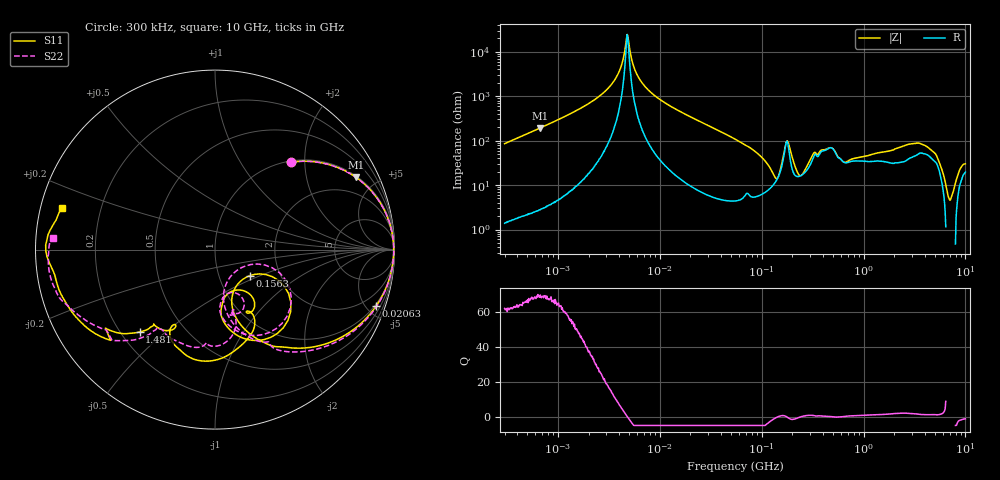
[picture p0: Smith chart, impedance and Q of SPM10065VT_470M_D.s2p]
! S-Parameter Data Generated by TDK Corporation
! Copyright(C) 2020 TDK Corporation.
! All Rights Reserved.
! TDK P/N: SPM10065VT-470M-D (Inductor)
! Property: L=47uH at 100kHz
! Size(LxWxT): 10.5x10x6.5mm
! Model Type: s2p (Touchstone File Format Version 1.0)
! Frequency: DC=Yes Start=0.3MHz Stop=10000MHz 802points Log-sweep
! Model Generated on Apr. 23, 2020
! Port Assignments:
!  1 ---@@@--- 2
! Applicable Conditions:
!  Temperature = 25 degC
!  DC Bias Current = 0 A
!  Small Signal Operation
! Terms and conditions regarding TDK Simulation Models
! (1)This simulation model is being provided solely for informational purposes. Please refer to the specifications of the products in terms of detailed characteristics of such products.
! (2)In no event shall TDK Corporation of any of its subsidiaries be liable for any loss or damage arising, directly or indirectly,
!  From any information contained in this simulation model, including, but not limited to loss or damages arising from any inaccuracies, omissions or errors in connection with such information.
! (3)Any and all copyrights on this simulation model are owned by TDK Corporation.
!  Duplication or redistribution of this simulation model without prior written permission from TDK Corporation is prohibited.
! (4)This simulation model is subject to any modification or change without any prior notice.
! (5)Neither TDK Corporation nor any of its subsidiaries shall make any warranty, express or implied,
!  Including but not limited to the correctness, implied warranties of merchantability and fitness for a particular purpose with respect to this simulation models.
! (6)The use of this simulation model shall be deemed to have consented to the terms and conditions hereof.
# Hz S MA R 50
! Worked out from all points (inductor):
!   801 points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, 300 kHz to 10 GHz, reference 50 ohm
!   read as one part in series: L = 45.1 uH near 318.3 kHz
!   highest Q = 68.7 at 671.9 kHz (marker M1), where L = 45.8 uH
!   self-resonance near 4.797 MHz
!   S11 on the Smith chart (normalised r, x): 300 kHz: 1.02, +1.71; 20.63 MHz: 0.87, -5.73; 156.3 MHz: 1.41, -0.43; 1.481 GHz: 0.28, -0.41; 10 GHz: 0.06, +0.13
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300000  0.6457 49.0  0.7537 -40.1  0.7537 -40.1  0.6452 48.9
671858  0.8829 27.1  0.4566 -62.1  0.4568 -62.1  0.8831 27.1
1713600  0.98 10.0  0.1775 -78.7  0.1775 -78.8  0.9802 9.9
3509086  0.9949 2.2  0.04728 -83.1  0.04713 -83.2  0.9951 2.1
4177486  0.9956 0.6  0.02114 -78.7  0.02121 -78.6  0.9958 0.5
4796912  0.9958 -0.6  0.004064 -6.5  0.004055 -6.5  0.9959 -0.8
6127430  0.9948 -2.9  0.03606 80.2  0.03604 80.1  0.995 -3.1
9671944  0.9887 -7.7  0.1101 79.5  0.11 79.5  0.9889 -8.0
2.063197e7  0.951 -19.4  0.2836 68.7  0.2835 68.7  0.9511 -20.2
5.477226e7  0.7469 -47.1  0.6376 39.4  0.6374 39.4  0.7439 -49.9
1.145169e8  0.3947 -72.9  0.856 4.8  0.8556 4.8  0.3857 -78.2
1.563148e8  0.2427 -36.6  0.7934 -21.3  0.793 -21.3  0.1756 -36.1
1.855783e8  0.5793 -57.5  0.5459 -1.6  0.5457 -1.6  0.5566 -52.5
2.320257e8  0.3346 -84.2  0.7955 -16.4  0.7952 -16.3  0.3393 -85.4
3.126428e8  0.2907 -53.7  0.6968 -42.8  0.6965 -42.8  0.3025 -60.7
3.970454e8  0.4999 -64.9  0.5404 -47.6  0.5401 -47.6  0.3748 -76.9
4.986356e8  0.6199 -91.8  0.4597 -45.9  0.4594 -45.9  0.4914 -79.1
7.84152e8  0.4913 -117.1  0.5127 -71.8  0.5126 -71.8  0.5519 -116.5
1.481453e9  0.6217 -132.5  0.3038 -128.4  0.3035 -128.4  0.6346 -129.6
1.767019e9  0.7045 -138.6  0.2209 -149.5  0.2208 -149.4  0.7141 -134.8
4.749267e9  0.9023 -169.3  0.02343 -169.5  0.02338 -169.3  0.9145 -164.7
1e10  0.8857 164.9  0.02735 140.9  0.02744 141.1  0.9036 175.9
